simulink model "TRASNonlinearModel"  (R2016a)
settings: Solver=VariableStepAuto  StartTime=0.0  StopTime=100.0  RelTol=1e-3
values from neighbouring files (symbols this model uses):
  a1 = 0.0135    [TRAS_Nonlinear_Parameters.m]
  a2 = 0.02    [TRAS_Nonlinear_Parameters.m]
  b1 = 0.0924    [TRAS_Nonlinear_Parameters.m]
  B1phi = 0.1    [TRAS_Nonlinear_Parameters.m]
  B1psi = 0.006    [TRAS_Nonlinear_Parameters.m]
  b2 = 0.09    [TRAS_Nonlinear_Parameters.m]
  B2psi = 0.001    [TRAS_Nonlinear_Parameters.m]
  I1 = 0.068    [TRAS_Nonlinear_Parameters.m]
  I2 = 0.02    [TRAS_Nonlinear_Parameters.m]
  K1 = 1.1    [TRAS_Nonlinear_Parameters.m]
  K2 = 0.8    [TRAS_Nonlinear_Parameters.m]
  Kc = -0.2    [TRAS_Nonlinear_Parameters.m]
  Kgy = 0.05    [TRAS_Nonlinear_Parameters.m]
  Mg = 0.32    [TRAS_Nonlinear_Parameters.m]
  T0 = 3.5    [TRAS_Nonlinear_Parameters.m]
  T10 = 1    [TRAS_Nonlinear_Parameters.m]
  T11 = 1.1    [TRAS_Nonlinear_Parameters.m]
  T20 = 1    [TRAS_Nonlinear_Parameters.m]
  T21 = 1    [TRAS_Nonlinear_Parameters.m]
  Tp = 2    [TRAS_Nonlinear_Parameters.m]

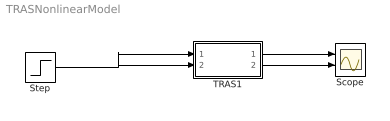
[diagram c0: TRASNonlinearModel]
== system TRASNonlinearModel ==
  Scope : Scope  NumInputPorts=2
  Step : Step  Time=0  SampleTime=0
  TRAS1 : Subsystem
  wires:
  Step/1 -> TRAS1/1(In1), TRAS1/2(In2)
  TRAS1/1(Out1) -> Scope/1
  TRAS1/2(Out2) -> Scope/2

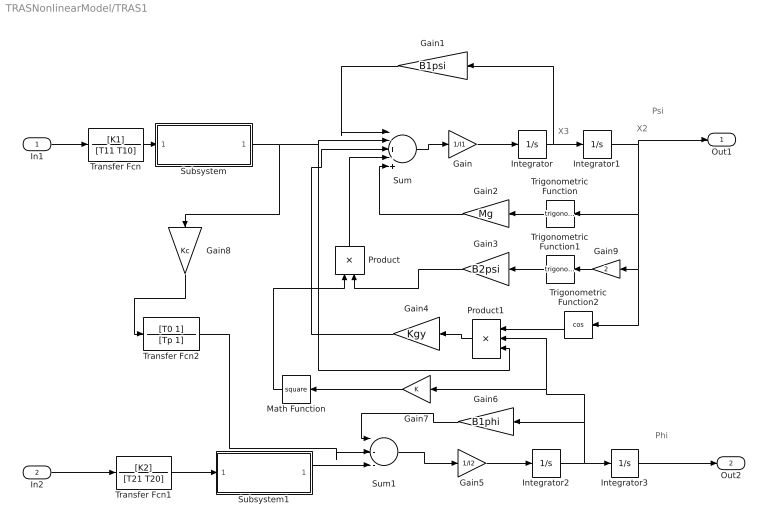
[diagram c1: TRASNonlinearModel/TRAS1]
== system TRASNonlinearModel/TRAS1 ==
  note: Phi
  note: Psi
  note: X3
  note: X2
  In1 : Inport
  In2 : Inport  Port=2
  Gain : Gain  Gain=1/I1
  Gain1 : Gain  Gain=B1psi
  Gain2 : Gain  Gain=Mg
  Gain3 : Gain  Gain=B2psi
  Gain4 : Gain  Gain=Kgy
  Gain5 : Gain  Gain=1/I2
  Gain6 : Gain  Gain=B1phi
  Gain7 : Gain
  Gain8 : Gain  Gain=Kc
  Gain9 : Gain  Gain=2
  Integrator{,1..3} (4 alike) : Integrator
  Math Function : Math  Operator=square
  Product : Product
  Product1 : Product  Inputs=3
  Subsystem : Subsystem
  Subsystem1 : Subsystem
  Sum : Sum  Inputs=|-+-+-
  Sum1 : Sum  Inputs=|--+
  Transfer Fcn : TransferFcn  Numerator=[K1]  Denominator=[T11 T10]
  Transfer Fcn1 : TransferFcn  Numerator=[K2]  Denominator=[T21 T20]
  Transfer Fcn2 : TransferFcn  Numerator=[T0 1]  Denominator=[Tp 1]
  Trigonometric Function : Trigonometry
  Trigonometric Function1 : Trigonometry
  Trigonometric Function2 : Trigonometry  Operator=cos
  Out1 : Outport
  Out2 : Outport  Port=2
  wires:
  In1/1 -> Transfer Fcn/1
  Transfer Fcn/1 -> Subsystem/1(In1)
  Sum/1 -> Gain/1
  Gain/1 -> Integrator/1
  Integrator/1 -> Gain1/1, Integrator1/1
  Integrator1/1 -> Gain9/1, Trigonometric Function2/1, Trigonometric Function/1, Out1/1
  Subsystem/1(M1) -> Gain8/1, Product1/3, Sum/2
  Gain1/1 -> Sum/1
  Gain2/1 -> Sum/5
  Gain3/1 -> Product/2
  Trigonometric Function/1 -> Gain2/1
  Trigonometric Function1/1 -> Gain3/1
  Product/1 -> Sum/4
  Trigonometric Function2/1 -> Product1/1
  Product1/1 -> Gain4/1
  Gain4/1 -> Sum/3
  In2/1 -> Transfer Fcn1/1
  Transfer Fcn1/1 -> Subsystem1/1(In1)
  Subsystem1/1(M1) -> Sum1/3
  Sum1/1 -> Gain5/1
  Gain5/1 -> Integrator2/1
  Integrator2/1 -> Gain7/1, Product1/2, Gain6/1, Integrator3/1
  Gain6/1 -> Sum1/1
  Gain7/1 -> Math Function/1
  Math Function/1 -> Product/1
  Gain8/1 -> Transfer Fcn2/1
  Transfer Fcn2/1 -> Sum1/2
  Integrator3/1 -> Out2/1
  Gain9/1 -> Trigonometric Function1/1

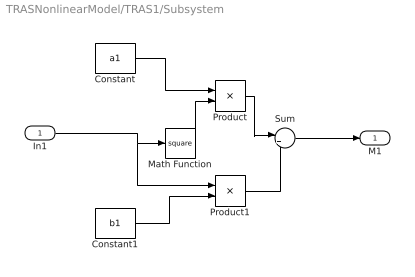
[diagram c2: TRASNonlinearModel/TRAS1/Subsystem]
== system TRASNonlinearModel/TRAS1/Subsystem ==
  In1 : Inport
  Constant : Constant  Value=a1
  Constant1 : Constant  Value=b1
  Math Function : Math  Operator=square
  Product : Product
  Product1 : Product
  Sum : Sum  Inputs=|++
  M1 : Outport
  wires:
  In1/1 -> Math Function/1, Product1/1
  Constant/1 -> Product/1
  Constant1/1 -> Product1/2
  Product/1 -> Sum/1
  Product1/1 -> Sum/2
  Sum/1 -> M1/1
  Math Function/1 -> Product/2

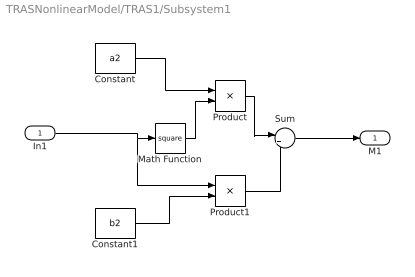
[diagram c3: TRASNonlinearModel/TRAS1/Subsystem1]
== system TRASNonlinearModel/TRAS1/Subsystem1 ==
  In1 : Inport
  Constant : Constant  Value=a2
  Constant1 : Constant  Value=b2
  Math Function : Math  Operator=square
  Product : Product
  Product1 : Product
  Sum : Sum  Inputs=|++
  M1 : Outport
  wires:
  In1/1 -> Product1/1, Math Function/1
  Constant/1 -> Product/1
  Constant1/1 -> Product1/2
  Product/1 -> Sum/1
  Product1/1 -> Sum/2
  Sum/1 -> M1/1
  Math Function/1 -> Product/2
